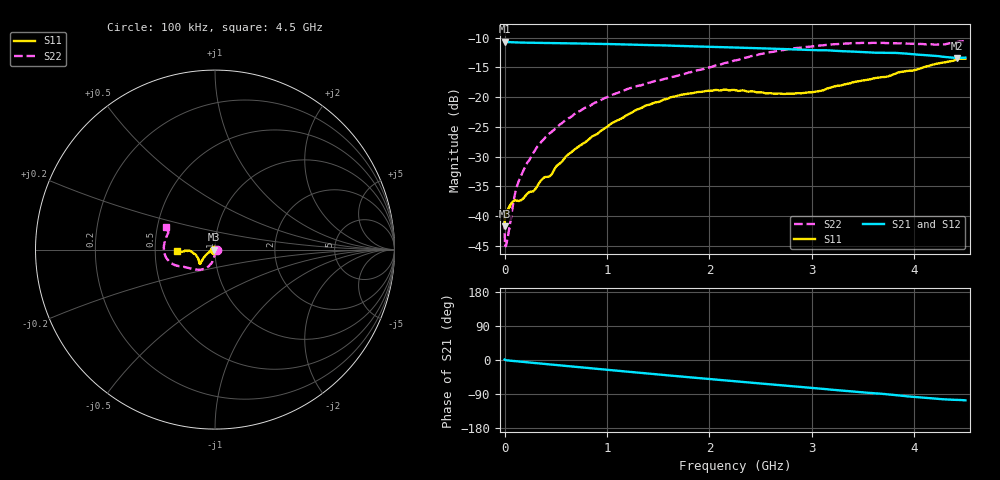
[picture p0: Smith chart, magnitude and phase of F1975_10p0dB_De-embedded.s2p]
! Integrated Device Technology
! Corporate Headquarters
! 6024 Silver Creek Valley Road
! San Jose, CA 95138  USA
! Phone:  1-408-284-8200
! Toll Free:  1-800-223-1366
! Webpage:  http://www.idt.com/
! Timing and RF Division
! 515 Groton Road, Suite 102
! Westford, MA 01886-6024
! Device:  F1975
! Description: 6-bit, 75 ohm, 0.5 dB Digital Step Attenuator
! Frequency:  5.0 MHz -  3.00 GHz
! Package:  4x4 mm QFN Plastic Package: 20 pin
! Ports:  2 RF, 11 DC
!  Pin  1  = D5 (16 dB)
!  Pin  2  = RF1  =  Port 1
!  Pin  3  = Serial Data In (DATA)
!  Pin  4  = Serial Clock (CLK)
!  Pin  5  = Serial Latch Enable (LE)
!  Pin  6  = VDD
!  Pin  7  = NC
!  Pin  8  = NC
!  Pin  9  = NC
!  Pin 10  = GND
!  Pin 11  = GND
!  Pin 12  = NC
!  Pin 13  = VMODE
!  Pin 14  = RF2  =  Port 2
!  Pin 15  = D4 (8 dB)
!  Pin 16  = D3 (4 dB)
!  Pin 17  = D2 (2 dB)
!  Pin 18  = NC
!  Pin 19  = D1 (1 dB)
!  Pin 20  = D0 (0.5 dB)
! State:  20
! Atten State:  10.0 dB
! Voltage:  +3.30 Volts
! Current:  0.596 mA
! Data:  The device was measured on a F1975 evaluation board which has
!  individual transmission lines to the RF pins.  Data was collected
!  using a calibrated network analyzer.  The evaluation board was
!  de-embedded using Automatic Fixture Removal (AFR).
!  The reference plane is the edge of the package pin.
! Misc:
!  Action Tracker AT0415
! Date Measured:  2018-02-08
! Date:  2018-03-26  MJV
! Note:
!  Integrated Device Technology supplies this data as a sample of measured
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# GHz S dB R 75
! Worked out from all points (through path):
!   291 points, 100 kHz to 4.5 GHz, reference 75 ohm
!   highest |S21| = -10.68 dB at 100 kHz (marker M1); lowest = -13.4 dB at 4.42 GHz (marker M2)
!   group delay of S21, straight-line fit = 67.2 ps
!   lowest |S11| = -41.7 dB at 100 kHz (marker M3), VSWR 1.02, Z = 73.8 - j0.0128 ohm
!   |S11| at or under -10 dB: start of sweep to end of sweep
!   |S22| runs from -45.1 to -10.5 dB; largest |S21 - S12| = 0.00015
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0.0001  -41.70 -179.4  -10.68 1.2  -10.68 1.2  -40.76 -2.1
0.0009  -40.88 -175.5  -10.71 1.0  -10.71 1.0  -42.95 -10.2
0.003  -40.45 -176.9  -10.72 0.7  -10.72 0.7  -44.38 -14.0
0.013  -39.71 -174.7  -10.75 -0.6  -10.75 -0.6  -45.05 -41.1
0.037  -38.80 -173.4  -10.77 -1.2  -10.77 -1.2  -43.07 -69.9
0.08  -37.54 -167.7  -10.80 -2.4  -10.80 -2.4  -38.29 -92.5
0.12  -37.41 -163.2  -10.82 -3.5  -10.82 -3.5  -35.01 -92.7
0.22  -36.26 -165.1  -10.85 -6.1  -10.85 -6.0  -31.05 -93.2
0.28  -35.85 -162.9  -10.87 -7.6  -10.87 -7.6  -29.40 -96.2
0.36  -33.92 -163.5  -10.89 -9.6  -10.89 -9.6  -27.47 -96.2
0.42  -33.41 -159.7  -10.91 -11.1  -10.91 -11.1  -26.40 -96.9
0.6  -29.95 -159.8  -10.96 -15.7  -10.96 -15.7  -23.78 -101.0
0.76  -27.89 -153.9  -11.00 -19.7  -11.00 -19.7  -22.07 -104.9
1.04  -24.46 -148.7  -11.09 -26.8  -11.09 -26.8  -19.70 -111.8
1.52  -20.70 -140.1  -11.28 -38.6  -11.28 -38.6  -17.15 -126.6
1.88  -19.17 -136.7  -11.49 -47.3  -11.48 -47.3  -15.51 -140.2
2.26  -18.86 -138.7  -11.67 -56.3  -11.67 -56.3  -13.80 -151.9
2.64  -19.46 -150.0  -11.87 -65.3  -11.87 -65.3  -12.33 -159.6
3.02  -19.13 -164.9  -12.10 -74.1  -12.09 -74.1  -11.44 -167.3
3.76  -16.43 -177.2  -12.55 -91.0  -12.54 -91.0  -10.92 173.4
4.42  -13.65 -175.8  -13.41 -105.3  -13.40 -105.3  -10.74 157.0
4.5  -13.53 -177.7  -13.37 -106.5  -13.36 -106.5  -10.48 155.7
